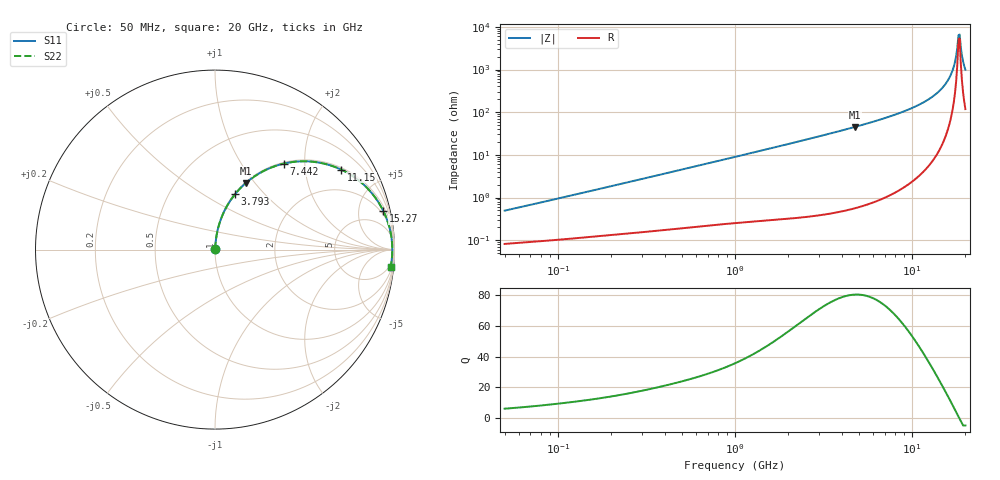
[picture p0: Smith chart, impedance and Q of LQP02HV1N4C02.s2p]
!Murata Part Number: LQP02HV1N4C02
!These Parameters are Measured in Series Mode Connection
!  o--[Z]--o
!Port1  Port2
!  o-------o
!Freq. Start=50[MHz] Stop=20[GHz], 401[Steps]
# Hz S RI R 50
!Freq.(Hz) S11(Real) S11(Imag) S21(Real) S21(Imag) S12(Real) S12(Imag) S22(Real) S22(Imag)
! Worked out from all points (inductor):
!   401 points, 50 MHz to 20 GHz, reference 50 ohm
!   read as one part in series: L = 1.53 nH near 51.52 MHz
!   highest Q = 80.4 at 4.748 GHz (marker M1), where L = 1.51 nH
!   self-resonance near 18.28 GHz
!   S11 on the Smith chart (normalised r, x): 50 MHz: 1.00, +0.01; 3.793 GHz: 1.01, +0.70; 7.442 GHz: 1.02, +1.57; 11.15 GHz: 1.07, +3.11; 15.27 GHz: 1.48, +8.61; 20 GHz: 3, -20
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5e7  0.000842 0.00485  0.9992 -0.00485  0.9992 -0.00485  0.000842 0.00485
1.364002e8  0.00131 0.0127  0.9987 -0.0127  0.9987 -0.0127  0.00131 0.0127
3.721004e8  0.00281 0.0336  0.9972 -0.0336  0.9972 -0.0336  0.00281 0.0336
1e9  0.0104 0.0884  0.9896 -0.0884  0.9896 -0.0884  0.0104 0.0884
2.728004e9  0.0606 0.2313  0.9394 -0.2313  0.9394 -0.2313  0.0606 0.2313
3.792786e9  0.1126 0.3097  0.8874 -0.3097  0.8874 -0.3097  0.1126 0.3097
4.748272e9  0.1715 0.3708  0.8285 -0.3708  0.8285 -0.3708  0.1715 0.3708
7.442007e9  0.3839 0.4793  0.6161 -0.4793  0.6161 -0.4793  0.3839 0.4793
9.316812e9  0.5499 0.489  0.4501 -0.489  0.4501 -0.489  0.5499 0.489
1.115139e10  0.7037 0.4457  0.2963 -0.4457  0.2963 -0.4457  0.7037 0.4457
1.334722e10  0.8524 0.3386  0.1476 -0.3386  0.1476 -0.3386  0.8524 0.3386
1.527346e10  0.9383 0.2145  0.0617 -0.2145  0.0617 -0.2145  0.9383 0.2145
1.621653e10  0.9643 0.1496  0.0357 -0.1496  0.0357 -0.1496  0.9643 0.1496
1.696185e10  0.9778 0.0982  0.0222 -0.0982  0.0222 -0.0982  0.9778 0.0982
1.747767e10  0.9837 0.063  0.0163 -0.063  0.0163 -0.063  0.9837 0.063
1.800918e10  0.987 0.0273  0.013 -0.0273  0.013 -0.0273  0.987 0.0273
1.828096e10  0.9877 0.0094  0.0123 -0.0094  0.0123 -0.0094  0.9877 0.0094
1.855685e10  0.9878 -0.00854  0.0122 0.00854  0.0122 0.00854  0.9878 -0.00854
1.88369e10  0.9872 -0.0265  0.0128 0.0265  0.0128 0.0265  0.9872 -0.0265
1.940974e10  0.984 -0.0621  0.016 0.0621  0.016 0.0621  0.984 -0.0621
1.970266e10  0.9815 -0.0798  0.0185 0.0798  0.0185 0.0798  0.9815 -0.0798
2e10  0.9783 -0.0974  0.0217 0.0974  0.0217 0.0974  0.9783 -0.0974
